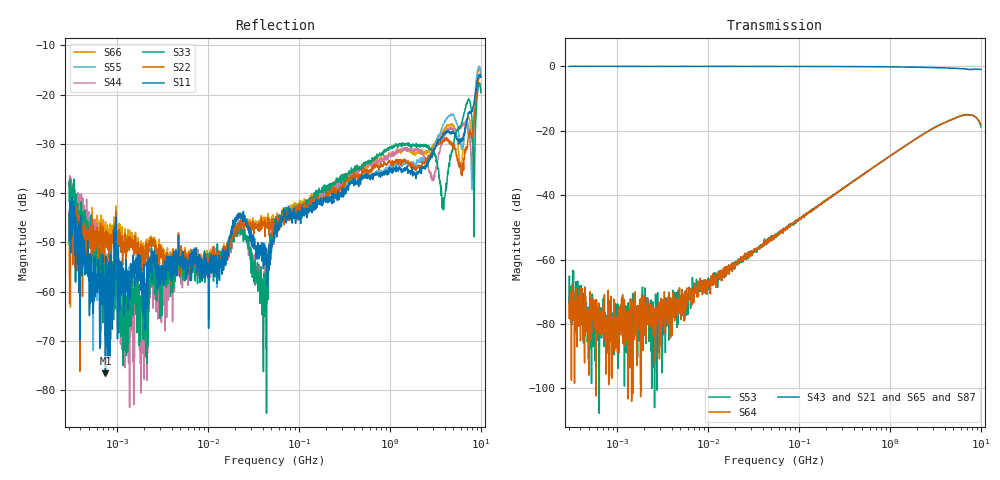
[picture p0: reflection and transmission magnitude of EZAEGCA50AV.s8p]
!*** S-Parameter ***
!Copyright (C)  Panasonic Industry
!ESD Suppressor Array
!Parts No.  EZAEGCA50AV
# Hz S dB R 50
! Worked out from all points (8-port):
!   1601 points, 300 kHz to 10 GHz, reference 50 ohm
!   strongest paths, dB at 300 kHz, 4.054 MHz, 54.77 MHz, 740.1 MHz, 10 GHz:
!     S43: 0.0, 0.0, 0.0, -0.1, -1.0
!     S21: 0.0, 0.0, 0.0, -0.1, -0.9
!     S65: 0.0, 0.0, 0.0, -0.1, -1.0
!     S87: 0.0, 0.0, 0.0, -0.1, -0.9
!     S64: -73.5, -73.0, -52.4, -30.4, -18.0
!     S53: -73.6, -75.4, -52.9, -30.5, -18.8
!   lowest |S11| = -76.6 dB at 751.1 kHz (marker M1), VSWR 1.00, Z = 50 - j0.0139 ohm
!   |S11| at or under -10 dB: start of sweep to end of sweep
